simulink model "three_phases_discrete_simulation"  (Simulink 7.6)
settings: Solver=ode15s  SolverMode=SingleTasking  StartTime=0.0  StopTime=1  MaxStep=5e-5  RelTol=1e-3  AbsTol=1e-2
libraries: powerlib x13, powerlib_extras x4

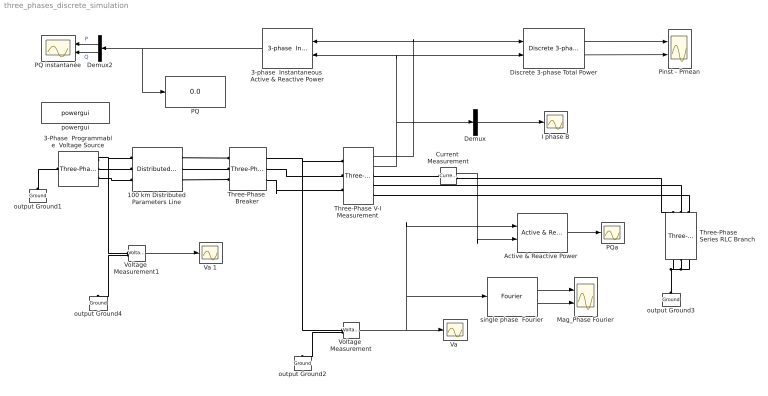
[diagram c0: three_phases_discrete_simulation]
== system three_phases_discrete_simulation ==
  100 km Distributed Parameters Line : powerlib/Elements/Distributed Parameters Line  DialogController=POWERSYS.PowerSysDialog  SystemSampleTime=-1  Phases=3  Frequency=60  Resistance=[0.01273 0.3864]  Inductance="[0.9337e-3  4.1264e-3]"  Capacitance=[12.74e-9 7.751e-9]  Length=100  x1=[0 -7.69769322013213e-013 8436.85546053586 -20317.9592956091;0.000113108313399149 -6.17501500960306e-013 9295.29862436812 -19939.8451218614;0.000226216626798297 -4.64111083875514e-013 10136.8432619058 -19525.4810102992;0.000339324940197446 -3.0987692914749e-013 10959.9594745669 -19075.6202603179;0.000452433253596594 -1.55079429050275e-013 11763.1508659981 -18591.0807029545;0.000565541566995742 0 1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  x2=[0 2.11533082169044e-008 4434.37379711385 -10546.8351944296;0.000113108313399149 2.13386198781741e-008 4879.93255874473 -10348.2202244207;0.000226216626798297 2.14851386782703e-008 5316.61977444771 -10130.7925536444;0.000339324940197446 2.15925982511626e-008 5743.64156220831 -9894.9474579664;0.000452433253596594 2.16608032391233e-008 6160.22161142046 -9641.11369548397;0.000565541566995742 2.168962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  x3=[0 2.44744185151026e-012 299.44583185442 46.797125708527;0.000113108313399149 8.10557095288358e-012 297.178777244067 59.5193375744307;0.000226216626798297 1.37489644110662e-011 294.371462058515 72.133345375927;0.000339324940197446 1.93673627350404e-011 291.028989898132 84.6162172900454;0.000452433253596594 2.49505518740642e-011 287.157437259864 96.9452598942508;0.000565541566995742 3.0488381786456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  x4=[0 2.47724302449986e-011 -259.473835604733 -163.493684175778;0.000113108313399149 1.94874414759606e-011 -252.268584577248 -174.405898306813;0.000226216626798297 1.41670252230404e-011 -244.604718126844 -185.001048642745;0.000339324940197446 8.82085381604484e-012 -236.496168893447 -195.259873572538;0.000452433253596594 3.4586464067459e-012 -227.957677934656 -205.163722912932;0.000565541566995742 -1.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  x5=0.000565541566995742  Measurements=None
  3-Phase  Programmable  Voltage Source : powerlib/Electrical Sources/Three-Phase Programmable Voltage Source  DialogController=POWERSYS.PowerSysDialog  SystemSampleTime=-1  PositiveSequence="[22e3 0  60]"  VariationEntity=Amplitude  VariationType=Step  VariationStep=2  VariationRate=10  VariationMagnitude=0.3  VariationFrequency=2  VariationTiming=[0.2 0.3]  VariationPhaseA=off  Amplitudes=[1 0.8 1.2 1.0]  TimeValues=[0 0.1 0.15 0.2]  HarmonicGeneration=off  HarmonicA=[5 0.08 -45 2]  HarmonicB=[2 0 0 2]  Timing="[0.1  1]"
  3-phase  Instantaneous  Active & Reactive Power : powerlib_extras/Measurements/3-phase  Instantaneous  Active & Reactive Power  DialogController=POWERSYS.PowerSysDialog  SystemSampleTime=-1
  "Active & Reactive Power " : powerlib_extras/Measurements/Active & Reactive Power  DialogController=POWERSYS.PowerSysDialog  SystemSampleTime=-1  f1=60
  Current  Measurement : powerlib/Measurements/Current Measurement  DialogController=POWERSYS.PowerSysDialog  SystemSampleTime=-1  PhasorSimulation=off  OutputType=Complex  PSBequivalent=0
  Demux : Demux  Outputs=3
  Demux2 : Demux  Outputs=2
  Discrete 3-phase Total Power : powerlib_extras/Discrete Measurements/Discrete 3-phase Total Power  DialogController=POWERSYS.PowerSysDialog  SystemSampleTime=-1  Freq=60  Par_Vinit=[0 0]  Par_Iinit=[0 0]  Ts=50e-6
  I phase B : Scope
  Mag_Phase Fourier : Scope  NumInputPorts=2
  PQ : Display
  PQ instantanée : Scope  NumInputPorts=2
  PQa : Scope
  Pinst - Pmean : Scope  NumInputPorts=2
  Three-Phase  Breaker : powerlib/Elements/Three-Phase Breaker  DialogController=POWERSYS.PowerSysDialog  SystemSampleTime=-1  InitialState=closed  SwitchA=on  SwitchB=on  SwitchC=on  SwitchTimes="[20/60  30/60]"  External=off  BreakerResistance=0.001  SnubberResistance=1e6  SnubberCapacitance=inf  Measurements=None
  Three-Phase Series RLC Branch : powerlib/Elements/Three-Phase Series RLC Branch  DialogController=POWERSYS.PowerSysDialog  PhysicalDomain=powersysdomain  SubClassName=unknown  LeftPortType=p1  RightPortType=p1  LConnTagsString=A|B|C  RConnTagsString=A|B|C  BranchType=RL  Resistance=1  Inductance=0.1  Capacitance=1.0  Measurements=None
  Three-Phase V-I Measurement : powerlib/Measurements/Three-Phase V-I Measurement  DialogController=POWERSYS.PowerSysDialog  SystemSampleTime=-1  VoltageMeasurement=phase-to-ground  SetLabelV=off  LabelV=V1  Vpu=on  VpuLL=off  CurrentMeasurement=yes  SetLabelI=off  LabelI=I1  Ipu=on  Pbase=10e6  Vbase=25e3  OutputType=Magnitude  PhasorSimulation=off  PSBequivalent=0
  "Va " : Scope
  Va 1 : Scope
  Voltage  Measurement : powerlib/Measurements/Voltage Measurement  DialogController=POWERSYS.PowerSysDialog  SystemSampleTime=-1  PhasorSimulation=off  OutputType=Complex  PSBequivalent=0
  Voltage  Measurement1 : powerlib/Measurements/Voltage Measurement  DialogController=POWERSYS.PowerSysDialog  SystemSampleTime=-1  PhasorSimulation=off  OutputType=Complex  PSBequivalent=0
  output Ground{1..4} (4 alike) : powerlib/Elements/Ground  DialogController=POWERSYS.PowerSysDialog  PhysicalDomain=powersysdomain  SubClassName=unknown  LeftPortType=p1  RightPortType=p1  LConnTagsString=a
  powergui : powerlib/powergui  Priority=2  SystemSampleTime=-1  SimulationMode=Discrete  SampleTime=1e-5  frequency=60  SPID=off  DisableSnubberDevices=off  DisableRonSwitches=off  DisableVfSwitches=off  SwTol=0  Interpol=off  frequencyindice=60  echomessages=off  HookPort=off  DisplayEquations=off  FunctionMessages=off  EnableUseOfTLC=off  x0status=blocks  RestoreLinks=warning  ResistiveCurrentMeasurement=off  Frange=[0:2:500]  Ylog=off  Xlog=off  ShowGrid=off  save=off  variable=ZData  ZoomFFT=on  StartTime=0.0  cycles=1  DisplayStyle=off  fundamental=60  FreqAxis=off  MaxFrequency=1000  frequencyindicesteady=1  RmsSteady=1  display=off  Ts=0  methode=off
  single phase  Fourier : powerlib_extras/Measurements/Fourier  DialogController=POWERSYS.PowerSysDialog  SystemSampleTime=-1  f1=60  n=1
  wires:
  3-phase  Instantaneous  Active & Reactive Power/1 -> Demux2/1, PQ/1
  Demux2/1 -> PQ instantanée/1  "P"
  Demux2/2 -> PQ instantanée/2  "Q"
  Voltage  Measurement/1 -> "Va "/1, single phase  Fourier/1, "Active & Reactive Power "/1
  single phase  Fourier/1 -> Mag_Phase Fourier/1
  single phase  Fourier/2 -> Mag_Phase Fourier/2
  Three-Phase V-I Measurement/1 -> 3-phase  Instantaneous  Active & Reactive Power/1, Discrete 3-phase Total Power/1
  Three-Phase V-I Measurement/2 -> 3-phase  Instantaneous  Active & Reactive Power/2, Discrete 3-phase Total Power/2, Demux/1
  Current  Measurement/1 -> "Active & Reactive Power "/2
  "Active & Reactive Power "/1 -> PQa/1
  Discrete 3-phase Total Power/1 -> Pinst - Pmean/1
  Discrete 3-phase Total Power/2 -> Pinst - Pmean/2
  Voltage  Measurement1/1 -> Va 1/1
  Demux/2 -> I phase B/1
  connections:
  3-Phase  Programmable  Voltage Source/RConn1 -- 100 km Distributed Parameters Line/LConn1 -- Voltage  Measurement1/LConn1
  3-Phase  Programmable  Voltage Source/RConn3 -- 100 km Distributed Parameters Line/LConn3
  output Ground1/LConn1 -- 3-Phase  Programmable  Voltage Source/LConn1
  Three-Phase  Breaker/RConn1 -- Voltage  Measurement/LConn1 -- Three-Phase V-I Measurement/LConn1
  100 km Distributed Parameters Line/RConn1 -- Three-Phase  Breaker/LConn1
  100 km Distributed Parameters Line/RConn2 -- Three-Phase  Breaker/LConn2
  100 km Distributed Parameters Line/RConn3 -- Three-Phase  Breaker/LConn3
  Voltage  Measurement/LConn2 -- output Ground2/LConn1
  3-Phase  Programmable  Voltage Source/RConn2 -- 100 km Distributed Parameters Line/LConn2
  Three-Phase  Breaker/RConn2 -- Three-Phase V-I Measurement/LConn2
  Three-Phase  Breaker/RConn3 -- Three-Phase V-I Measurement/LConn3
  Three-Phase Series RLC Branch/LConn2 -- Three-Phase V-I Measurement/RConn2
  Three-Phase Series RLC Branch/LConn3 -- Three-Phase V-I Measurement/RConn3
  Three-Phase V-I Measurement/RConn1 -- Current  Measurement/LConn1
  Current  Measurement/RConn1 -- Three-Phase Series RLC Branch/LConn1
  Three-Phase Series RLC Branch/RConn2 -- Three-Phase Series RLC Branch/RConn1 -- output Ground3/LConn1 -- Three-Phase Series RLC Branch/RConn3
  Voltage  Measurement1/LConn2 -- output Ground4/LConn1
